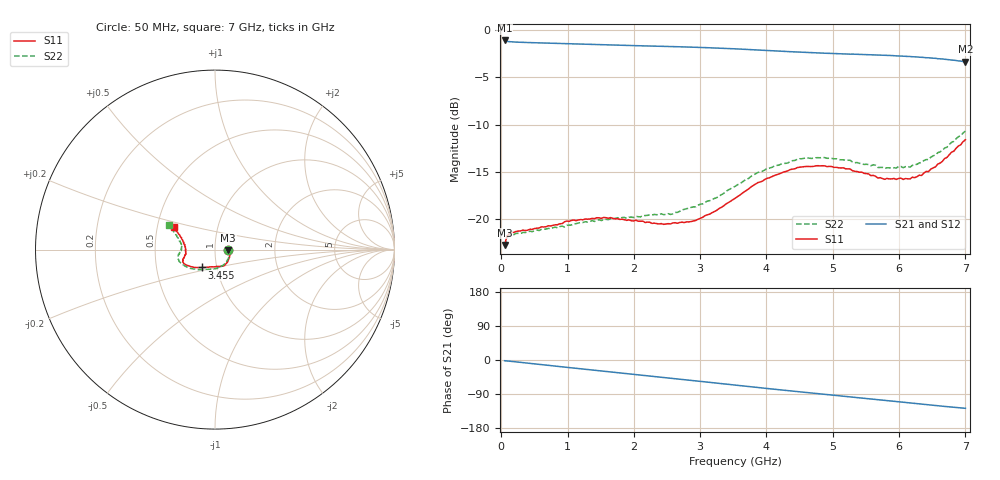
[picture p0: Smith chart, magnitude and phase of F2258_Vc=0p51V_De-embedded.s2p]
! Integrated Device Technology
! Corporate Headquarters
! 6024 Silver Creek Valley Road
! San Jose, CA 95138  USA
! Phone:  1-408-284-8200
! Toll Free:  1-800-223-1366
! Webpage:  http://www.idt.com/
! Timing and RF Division
! 515 Groton Road, Suite 102
! Westford, MA 01886-6024
! Device:  F2258
! Description: Voltage Variable RF Attenuator
! Frequency:  50.0 -  6000.00 MHz
! Package:  3x3 mm Thin QFN Plastic Package: 16 pin
! Ports:  2 RF, 2 DC
!  Pin  1  = NC
!  Pin  2  = NC
!  Pin  3  = RF2  = Port 2
!  Pin  4  = GND
!  Pin  5  = Vdd
!  Pin  6  = NC
!  Pin  7  = VCTRL
!  Pin  8  = NC
!  Pin  9  = GND
!  Pin 10  = RF1  = Port 1
!  Pin 11  = NC
!  Pin 12  = NC
!  Pin 13  = NC
!  Pin 14  = NC
!  Pin 15  = NC
!  Pin 16  = NC
! Vcntrl:  0.510 Volts
! Vdd:  +3.300 Volts
! Current:  1.103 mA
! Data:  The device was measured on a the F2258 evaluation board which has
!  individual transmission lines to the RF pins.  Data was collected
!  using a calibrated network analyzer.  The evaluation board was
!  de-embedded using a TRL calibration technique.
!  The reference plane is the edge of the package pin.
! Misc:  SN 10
!  Action Tracker AT0285
! Date Measured:  2014-12-10
! Date:  2016-01-13  MJV
! Note:
!  Integrated Device Technology supplies this data as a sample of measured
!  data at the package pin for this product.  Your particular data for this
!  product may vary.
!  Data was taken at 25 degrees C.
!  Integrated Device Technology reserves the right to change this data at anytime.
!Freq_(GHz)  S11M_(dB)  S11P_(deg)  S21M_(dB)  S21P_(deg)  S12M_(dB)  S12P_(deg)  S22M_(dB)  S22P_(deg)
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# GHz S dB R 50
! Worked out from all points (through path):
!   201 points, 50 MHz to 7 GHz, reference 50 ohm
!   highest |S21| = -1.11 dB at 50 MHz (marker M1); lowest = -3.4 dB at 7 GHz (marker M2)
!   group delay of S21, straight-line fit = 50.5 ps
!   lowest |S11| = -22.7 dB at 50 MHz (marker M3), VSWR 1.16, Z = 57.9 - j0.452 ohm
!   |S11| at or under -10 dB: start of sweep to end of sweep
!   |S22| runs from -22.8 to -10.7 dB; largest |S21 - S12| = 0.0004
!   S11 on the Smith chart (normalised r, x): 50 MHz: 1.16, -0.01; 3.455 GHz: 0.84, -0.17; 7 GHz: 0.61, +0.17
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0.05  -22.68 -3.0  -1.11 -2.0  -1.11 -2.0  -22.82 -3.0
0.08475  -21.79 -4.9  -1.20 -2.5  -1.20 -2.5  -21.94 -4.9
0.15425  -21.35 -7.7  -1.26 -3.7  -1.26 -3.7  -21.59 -8.5
0.71025  -20.67 -31.6  -1.40 -14.1  -1.40 -14.1  -20.94 -35.2
1.2315  -20.04 -51.7  -1.51 -23.8  -1.51 -23.8  -20.33 -58.8
1.6485  -19.81 -62.7  -1.59 -31.5  -1.59 -31.5  -19.94 -71.9
2.37825  -20.48 -82.0  -1.72 -44.8  -1.72 -44.8  -19.48 -90.4
2.552  -20.48 -87.7  -1.75 -48.0  -1.75 -48.0  -19.47 -95.8
2.93425  -20.11 -104.1  -1.84 -55.1  -1.84 -55.1  -18.67 -109.4
3.247  -19.05 -117.8  -1.91 -61.0  -1.91 -61.0  -17.71 -121.8
3.4555  -18.09 -127.1  -1.98 -64.9  -1.98 -64.9  -16.77 -129.5
3.525  -17.78 -129.5  -2.00 -66.2  -2.00 -66.2  -16.51 -132.6
4.0115  -15.66 -145.0  -2.18 -75.3  -2.18 -75.3  -14.63 -148.6
4.46325  -14.54 -154.3  -2.34 -83.4  -2.34 -83.4  -13.66 -160.1
4.7065  -14.40 -157.6  -2.41 -87.7  -2.41 -87.7  -13.55 -164.4
5.2625  -14.68 -164.3  -2.56 -97.4  -2.57 -97.4  -13.76 -172.8
5.6795  -15.63 -170.5  -2.65 -104.6  -2.65 -104.6  -14.52 -178.5
5.85325  -15.73 -174.7  -2.70 -107.7  -2.70 -107.7  -14.56 176.9
6.166  -15.72 177.2  -2.81 -113.3  -2.81 -113.3  -14.48 170.8
6.33975  -15.36 170.5  -2.89 -116.4  -2.89 -116.4  -13.98 166.3
6.722  -13.46 157.5  -3.12 -123.1  -3.12 -123.1  -12.38 157.1
7  -11.59 151.2  -3.37 -127.4  -3.37 -127.4  -10.68 152.0
